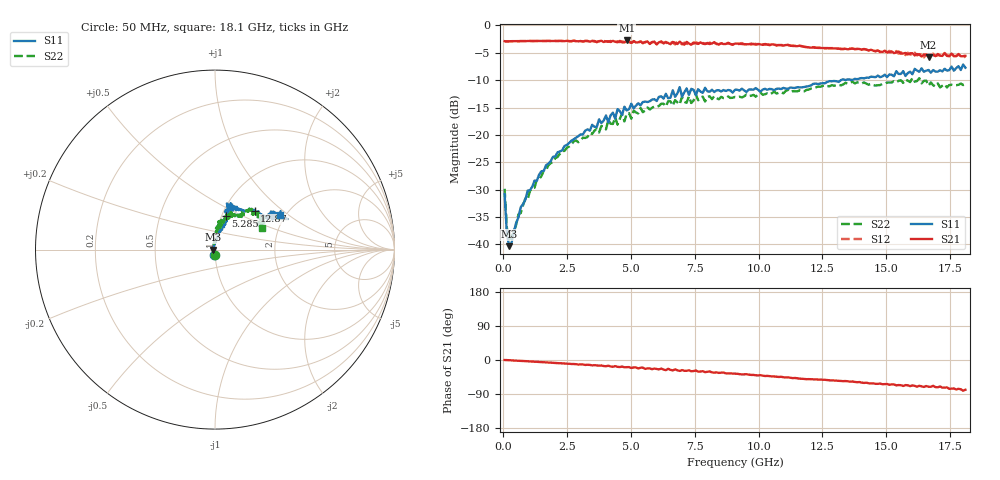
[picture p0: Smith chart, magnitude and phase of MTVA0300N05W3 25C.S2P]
! Network Analyzer HP8720D.06.14 Serial No. US36140669
!  7 Jul 2005  09:06:53
! Frequency  S11  S21  S12  S22
# HZ  S  DB R 50
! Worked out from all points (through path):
!   201 points, 50 MHz to 18.1 GHz, reference 50 ohm
!   highest |S21| = -2.76 dB at 4.833 GHz (marker M1); lowest = -5.7 dB at 16.66 GHz (marker M2)
!   group delay of S21, straight-line fit = 12 ps
!   lowest |S11| = -40.3 dB at 230.5 MHz (marker M3), VSWR 1.02, Z = 49 - j0.0574 ohm
!   |S11| at or under -10 dB: start of sweep to 13.23 GHz
!   |S22| runs from -39.1 to -9.6 dB; largest |S21 - S12| = 0.043
!   S11 on the Smith chart (normalised r, x): 50 MHz: 0.98, -0.06; 5.285 GHz: 1.05, +0.40; 12.87 GHz: 1.38, +0.66; 18.1 GHz: 1.88, +0.87
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5e7  -30.78 -104.4  -2.89 -0.0  -2.92 0.2  -29.84 -87.6
1.4025e8  -38.14 -138.8  -2.94 -0.3  -2.93 -0.3  -37.02 -139.7
2.305e8  -40.32 -176.5  -2.91 -0.5  -2.90 -0.6  -39.09 -173.3
9.525e8  -30.19 95.3  -2.86 -3.4  -2.85 -3.3  -31.75 106.6
1.76475e9  -25.28 84.7  -2.83 -6.7  -2.85 -6.8  -25.55 90.9
3.1185e9  -19.91 75.9  -2.94 -11.7  -2.95 -12.2  -20.51 87.4
4.743e9  -14.86 70.8  -3.13 -19.2  -3.06 -17.9  -17.55 79.7
4.83325e9  -15.53 76.1  -2.76 -18.8  -3.02 -19.8  -16.10 73.1
5.2845e9  -14.23 72.3  -3.09 -22.4  -3.17 -21.6  -16.08 72.4
6.09675e9  -13.05 69.0  -3.09 -24.9  -2.99 -24.4  -14.72 71.7
6.7285e9  -13.05 75.2  -3.19 -24.6  -3.49 -25.8  -13.65 65.5
6.909e9  -11.28 71.4  -2.97 -28.8  -3.11 -26.6  -14.44 65.7
6.99925e9  -13.00 71.5  -3.31 -26.6  -3.47 -29.1  -13.01 65.8
7.17975e9  -11.52 75.6  -3.02 -28.5  -3.36 -27.0  -14.14 61.7
7.54075e9  -12.74 67.6  -3.29 -27.6  -3.11 -31.0  -12.57 68.6
9.075e9  -11.76 67.2  -3.34 -36.0  -3.31 -36.1  -13.07 58.8
1.21435e10  -10.67 49.9  -4.03 -50.8  -3.97 -50.8  -11.44 53.1
1.28655e10  -10.22 44.4  -4.17 -53.7  -4.15 -53.9  -10.94 49.4
1.512175e10  -8.96 29.6  -4.92 -65.4  -4.66 -64.8  -10.43 42.5
1.6295e10  -8.47 27.4  -5.33 -68.0  -5.28 -72.0  -9.64 33.5
1.6656e10  -8.15 29.8  -5.75 -70.6  -5.51 -68.1  -11.01 29.3
1.81e10  -7.73 27.9  -5.57 -78.5  -5.89 -78.5  -10.79 24.2
